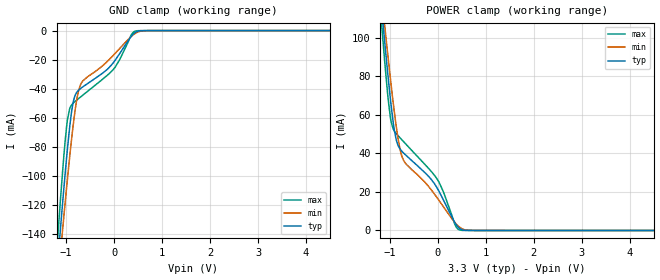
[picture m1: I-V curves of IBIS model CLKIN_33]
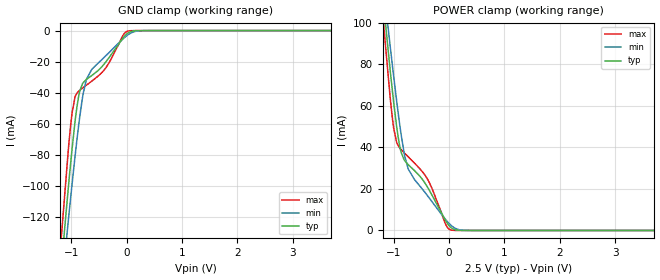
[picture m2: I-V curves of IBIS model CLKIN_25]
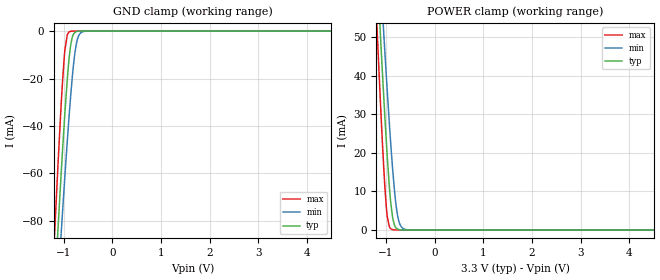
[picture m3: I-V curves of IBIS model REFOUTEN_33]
| Texas Instruments Incorporated
| Ultra-low Jitter LVCMOS Fanout Buffer/Level Translator w/ Universal Input
| Marketing part#   Voltage Range   Package-type   #pins/pkg drawing
| LMK00101   1.425V - 3.465V   LLP   32-pin SQ
[IBIS Ver]   4.1
[File name]   lmk00101.ibs
[File Rev]   1.1
[Date]   6/27/2014
[Source]   Model built from spectre simulations at:
   Texas Instruments Incorporated.
   Analog-eLab, HPA
   12500 TI Blvd
   Dallas, TX -75243
   For Support e-mail: elab_ibis@list.ti.com
[Notes]   Revision History
   Rev 1.1: 06/27/2014
   - Update Package Model
   Rev 1.0: 3/14/2012
   - ccomp values are based on PVT settings:
   WEAK: Low Voltage, High Temperature, Weak Process
   NOM: Nominal Voltage, Nominal Temperature, Nominal Process
   STRONG: High Voltage, Low Temperature, Fast Process
   - User may change ccomp in the order of number values as
   per end simulator used
   - C_comp although listed in numberical order of value are obtained from varying PVT conditions.
   For PVT conditions for each specific value, refer to the buffer description under repective [Model].
   IBIS model user is responsible for using appropriate C_comp to simulate for Signal Integrity.
[Disclaimer]  This model is designed as an aid for customers of Texas Instruments
 TI and its licensors and suppliers make no warranties, either expressed
 or implied, with respect to this  model, including the warranties of
 merchantability or fitness for a particular purpose.
 The model is provided solely on an "as is" basis. The entire risk as to
 its quality and performance is with the customer.
[Copyright] (C)Copyright 2014 Texas Instruments Incorporated.
   All rights reserved.
[Component]   LMK00101SQ
[Manufacturer]  Texas Instruments Incorporated
[Package]   |32-pin LLP SQ package
|   typ   min   max
R_pkg   0.4957   0.4512   0.5499
L_pkg   1.9075n   1.6913n   2.1938n
C_pkg   0.2495p   0.2380p   0.2608p
[Pin]   signal_name   model_name   R_pin   L_pin   C_pin
1   CLKout0   CMOSOUT   0.5458   2.1833n   0.2530p
2   Vddo   POWER   0.5111   1.9584n   0.2600p
3   CLKout1   CMOSOUT   0.4757   1.7915n   0.2461p
4   GND   GND   0.4554   1.7080n   0.2383p
5   CLKout2   CMOSOUT   0.4575   1.7023n   0.2381p
6   Vddo   POWER   0.4729   1.7891n   0.2459p
7   CLKout3   CMOSOUT   0.5049   1.9504n   0.2605p
8   CLKout4   CMOSOUT   0.5426   2.1789n   0.2535p
9   GND   GND   0.5435   2.1835n   0.2535p
10   Vddo   POWER   0.5093   1.9579n   0.2603p
11   OSCin   NC   0.4776   1.7944n   0.2465p
12   OSCout   NC   0.4584   1.7092n   0.2389p
13   CLKin0   CLKIN   0.4578   1.7109n   0.2389p
14   CLKin0*   CLKIN   0.4743   1.7979n   0.2468p
15   GND   GND   0.5087   1.9612n   0.2608p
16   GND   GND   0.5464   2.1841n   0.2534p
17   CLKout5   CMOSOUT   0.5364   2.1711n   0.2533p
18   CLKout6   CMOSOUT   0.5024   1.9433n   0.2602p
19   Vddo   POWER   0.4683   1.7789n   0.2456p
20   CLKout7   CMOSOUT   0.4520   1.6928n   0.2381p
21   GND   GND   0.4512   1.6913n   0.2380p
22   CLKout8   CMOSOUT   0.4690   1.7712n   0.2460p
23   Vddo   POWER   0.5059   1.9466n   0.2599p
24   CLKout9   CMOSOUT   0.5405   2.1711n   0.2529p
25   GND   GND   0.5470   2.1754n   0.2533p
26   GND   GND   0.5162   1.9557n   0.2604p
27   CLKin1*   CLKIN   0.4749   1.7838n   0.2465p
28   CLKin1   CLKIN   0.4562   1.7088n   0.2390p
29   SEL1   REFOUTEN   0.4580   1.7168n   0.2388p
30   SEL0   REFOUTEN   0.4814   1.8071n   0.2458p
31   OE   REFOUTEN   0.5115   1.9705n   0.2593p
32   GND   GND   0.5499   2.1938n   0.2525p
[Package Model] llp48_lmk00101
[Diff pin]  inv_pin  vdiff  tdelay_typ  tdelay_min  tdelay_max
13   14   0.15   NA  NA  NA   | Diff-in
27   28   0.15   NA  NA  NA   | Diff-in
| Model Selector Statements
[Model Selector]   CMOSOUT
CMOSOUT_33   3.3 volt Vcc
CMOSOUT_25   2.5 volt Vcc
CMOSOUT_18   1.8 volt Vcc
CMOSOUT_15   1.5 volt Vcc
[Model Selector]   CLKIN
CLKIN_33   3.3 volt Vcc
CLKIN_25   2.5 volt Vcc
[Model Selector]   REFOUTEN
REFOUTEN_33   3.3 volt Vcc
REFOUTEN_25   2.5 volt Vcc
[Define Package Model]  llp48_lmk00101
[Manufacturer]  Unknown
[OEM]  Unknown
[Description] Package Electrical model @ 2GHz, Buildsheet AD#LMK00101SQ-02
[Number Of Pins]  32
[Pin Numbers]
1   | L1:1
2   | L2:2
3   | L3:3
4   | L4:4
5   | L5:5
6   | L6:6
7   | L7:7
8   | L8:8
9   | L9:9
10   | L10:10
11   | L11:11
12   | L12:12
13   | L13:13
14   | L14:14
15   | L15:15
16   | L16:16
17   | L17:17
18   | L18:18
19   | L19:19
20   | L20:20
21   | L21:21
22   | L22:22
23   | L23:23
24   | L24:24
25   | L25:25
26   | L26:26
27   | L27:27
28   | L28:28
29   | L29:29
30   | L30:30
31   | L31:31
32   | L32:32
[Model Data]
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[End Model Data]
[End Package Model]
| Models and submodels in the file (8): CLKIN_33 (Input), CLKIN_25 (Input), REFOUTEN_33 (Input), REFOUTEN_25 (Input), CMOSOUT_33 (3-state), CMOSOUT_25 (3-state), CMOSOUT_18 (3-state), CMOSOUT_15 (3-state)
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|   Model   CLKIN_33
[Model]   CLKIN_33
Model_type   Input
Vinl = 1.2
Vinh = 1.35
|   typ   min   max
C_comp   0.334pF   0.334pF   0.334pF
[Voltage Range]   3.3   3.135   3.465
[Temperature Range]   45   125   -40
[Power Clamp Reference]   3.3   3.135   3.465
[GND Clamp Reference]   0   0   0
[GND Clamp]
|   Voltage   I(typ)   I(min)   I(max)
-3.3V     -1.09A     -1.005A    -1.209A
-1.181V   -161.9mA   -176.1mA   -145.1mA
-1.112V   -133.8mA   -150.8mA   -113.6mA
-1.063V   -114.4mA   -133.1mA   -92.33mA
-973.5mV  -81.6mA    -102.4mA   -61.43mA
-924mV    -65.73mA   -86.22mA   -53.42mA
-854.7mV  -49.53mA   -65.51mA   -49.97mA
-775.5mV  -42.3mA    -46.87mA   -47.7mA
-706.2mV  -40.03mA   -37.76mA   -45.84mA
-3.3mV    -21.51mA   -16.54mA   -26.2mA
432.3mV   -1.452mA   -2.108mA   -480.3uA
6.59V     0A         0A         0A
[POWER Clamp]
|   Voltage   I(typ)   I(min)   I(max)
-3.3V     736.4mA    674.6mA    821.9mA
-1.181V   117.5mA    123.9mA    109.8mA
-1.112V   98.9mA     107.2mA    88.87mA
-1.033V   78.62mA    88.68mA    67.5mA
-973.5mV  64.71mA    75.35mA    56.32mA
-864.6mV  46.64mA    53.42mA    50.15mA
-745.8mV  40.96mA    38.21mA    46.9mA
-13.2mV   21.94mA    16.89mA    26.59mA
353.1mV   4.136mA    4.187mA    3.278mA
442.2mV   1.233mA    1.901mA    362.3uA
768.9mV   12.13uA    18.74uA    12.42uA
6.59V     0A         0A         0A
|   Model   CLKIN_25
[Model]   CLKIN_25
Model_type   Input
Vinl = 1.2
Vinh = 1.35
|   typ   min   max
C_comp   0.334pF   0.334pF   0.334pF
[Voltage Range]   2.5   2.375   2.625
[Temperature Range]   45   125   -40
[Power Clamp Reference]   2.5   2.375   2.625
[GND Clamp Reference]   0   0   0
[GND Clamp]
|   Voltage   I(typ)   I(min)   I(max)
-2.5V     -725.6mA   -679.9mA   -791.5mA
-1.202V   -161.3mA   -176.9mA   -143.6mA
-1.052V   -101.3mA   -122.6mA   -76.94mA
-985mV    -76.47mA   -99.12mA   -53.21mA
-932.5mV  -59.17mA   -81.68mA   -43.03mA
-842.5mV  -38.65mA   -54.68mA   -38.4mA
-782.5mV  -33.58mA   -40.42mA   -36.72mA
-722.5mV  -31.41mA   -31.13mA   -35.12mA
-377.5mV  -20.35mA   -16.34mA   -24.16mA
5mV       -2.198mA   -3.271mA   -592.4uA
320mV     -13.02uA   -40.95uA   -11.33uA
4.992V    0A         0A         0A
[POWER Clamp]
|   Voltage   I(typ)   I(min)   I(max)
-2.5V     490.4mA    456.1mA    539mA
-1.21V    116.1mA    123.9mA    107.4mA
-1.067V   78.13mA    89.7mA     65.02mA
-1V       61.58mA    74.11mA    49.22mA
-947.5mV  50.14mA    62.54mA    42.5mA
-865mV    37.61mA    46.04mA    38.96mA
-737.5mV  31.69mA    29.61mA    35.52mA
-377.5mV  20.35mA    16.34mA    24.17mA
-62.5mV   4.828mA    5.299mA    3.016mA
12.5mV    1.975mA    3.072mA    479.7uA
320mV     14.63uA    42.46uA    13uA
4.992V    0A         0A         0A
|   Model REFOUTEN_33
[Model]   REFOUTEN_33
Model_type   Input
Vinl = 0.4
Vinh = 1.6
|   typ   min   max
C_comp   0.3093pF   0.3093pF   0.3093pF
[Voltage Range]   3.3   3.135   3.465
[Temperature Range]   45   125   -40
[Power Clamp Reference]   3.3   3.135   3.465
[GND Clamp Reference]   0   0   0
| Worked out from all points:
|   GND clamp passes 1 mA (typ) near -0.79 V on its own axis
|   POWER clamp passes 1 mA (typ) near -0.82 V on its own axis
[GND Clamp]
|   Voltage   I(typ)   I(min)   I(max)
-3.3V     -965.6mA   -893.6mA   -1.069A
-1.181V   -108.3mA   -129.3mA   -84.35mA
-1.112V   -82.59mA   -106mA     -55.39mA
-1.043V   -57.82mA   -83.32mA   -28.72mA
-973.5mV  -34.81mA   -61.42mA   -8.124mA
-924mV    -20.4mA    -46.56mA   -1.597mA
-884.4mV  -11.09mA   -35.36mA   -347uA
-825mV    -2.889mA   -20.4mA    -26.1uA
-745.8mV  -310.8uA   -6.404mA   -528.4nA
-676.5mV  -33.31uA   -1.499mA   -14.52nA
-577.5mV  -943.1nA   -148.2uA   0A
6.59V     0A         0A         0A
[POWER Clamp]
|   Voltage   I(typ)   I(min)   I(max)
-3.3V     638.8mA    590.5mA    708.3mA
-1.191V   69.15mA    82.63mA    53.96mA
-1.181V   66.68mA    80.4mA     51.15mA
-1.102V   47.28mA    62.82mA    29.5mA
-1.033V   31.21mA    47.91mA    12.87mA
-993.3mV  22.67mA    39.68mA    5.73mA
-933.9mV  11.5mA     27.94mA    888.7uA
-864.6mV  3.112mA    15.73mA    67.37uA
-805.2mV  711.5uA    7.563mA    4.089uA
-745.8mV  145.3uA    2.701mA    212.4nA
-577.5mV  412.5nA    72uA       0A
6.59V     0A         0A         0A
